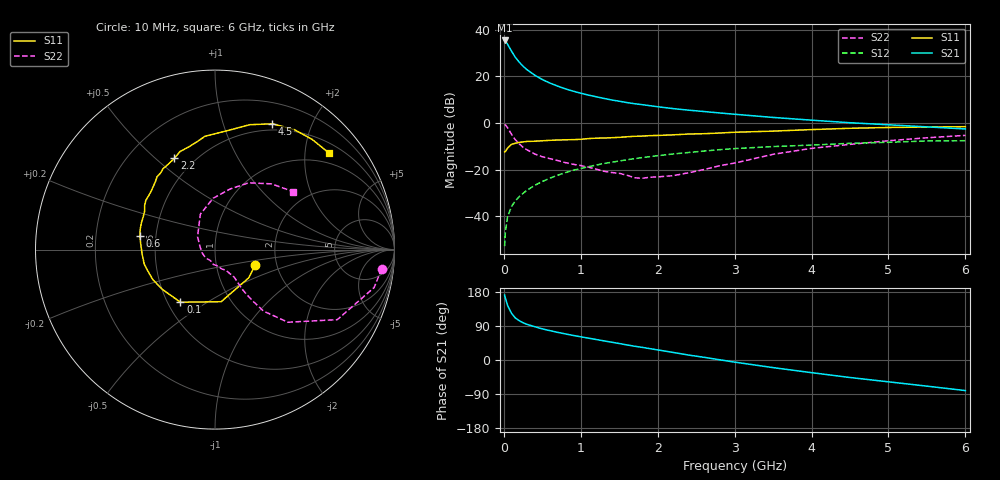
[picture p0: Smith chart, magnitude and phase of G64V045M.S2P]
! SIEMENS Small Signal Semiconductors
! BFG193
! Si NPN RF Bipolar Junction Transistor in SOT223
! VCE = 4 V  IC = 45 mA
! Common Emitter S-Parameters:  August  1996
# GHz  S  MA  R  50
!  f  S11  S21  S12  S22
! GHz  MAG  ANG  MAG  ANG  MAG  ANG  MAG  ANG
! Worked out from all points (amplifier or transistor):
!   36 points, 10 MHz to 6 GHz, reference 50 ohm
!   highest |S21| = 35.4 dB at 10 MHz (marker M1)
!   |S21| within 3 dB of that: start of sweep to 72.4 MHz
!   unconditionally stable (mu >= 1): 468.3 MHz to 2.381 GHz
!   at 250 MHz: K = 0.90, MSG = 27.2 dB, |S12| = -30.1 dB
!   at 1.4 GHz: K = 1.04, MAG = 12.1 dB, |S12| = -16.8 dB
!   at 6 GHz: K = 0.89, MSG = 2.5 dB, |S12| = -7.6 dB
!   S11 on the Smith chart (normalised r, x): 10 MHz: 1.55, -0.28; 100 MHz: 0.58, -0.39; 600 MHz: 0.41, +0.08; 2.2 GHz: 0.39, +0.58; 4.5 GHz: 0.43, +1.47; 6 GHz: 0.73, +2.56
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0.01  0.2396 -21.0  58.56 171.3  0.0023 86.9  0.935 -6.6
0.02  0.245 -40.1  56.43 163.7  0.0047 80.9  0.9115 -13.4
0.05  0.2924 -83.3  48.15 143.2  0.0101 71.9  0.7853 -29.8
0.1  0.3506 -123.3  34.48 123.3  0.0163 66.0  0.5733 -44.9
0.15  0.3676 -142.9  25.44 110.8  0.0215 65.7  0.4371 -51.7
0.2  0.3845 -154.0  20.11 103.8  0.0264 67.4  0.3585 -53.6
0.25  0.3932 -162.7  16.41 98.3  0.0312 68.0  0.3002 -54.9
0.3  0.4025 -168.4  13.91 94.1  0.0362 68.5  0.267 -55.5
0.4  0.407 -176.7  10.6 88.0  0.046 68.9  0.2176 -55.3
0.5  0.4157 175.2  8.521 82.1  0.0558 67.8  0.1891 -55.1
0.6  0.4257 169.6  7.151 77.5  0.0659 67.2  0.1719 -56.2
0.7  0.4317 164.9  6.164 72.9  0.076 65.8  0.1567 -58.4
0.8  0.4363 160.0  5.386 68.8  0.0865 63.9  0.1416 -60.2
1.1  0.4632 147.8  3.953 57.7  0.1158 58.8  0.1135 -71.2
1.3  0.476 140.9  3.362 50.5  0.1356 54.7  0.0925 -79.9
1.6  0.5062 130.7  2.736 39.8  0.163 48.1  0.0761 -102.5
2.2  0.5567 114.0  2.034 20.0  0.217 34.5  0.0744 -167.2
2.8  0.609 99.5  1.642 0.8  0.2678 20.6  0.121 143.5
3.5  0.6697 83.3  1.315 -20.1  0.3125 3.4  0.2134 112.5
4.5  0.7704 65.5  1.013 -46.2  0.3665 -16.6  0.348 76.0
5.5  0.8184 48.6  0.826 -69.0  0.4119 -39.9  0.4825 49.4
6  0.833 40.1  0.745 -80.7  0.4174 -53.3  0.5429 36.5
